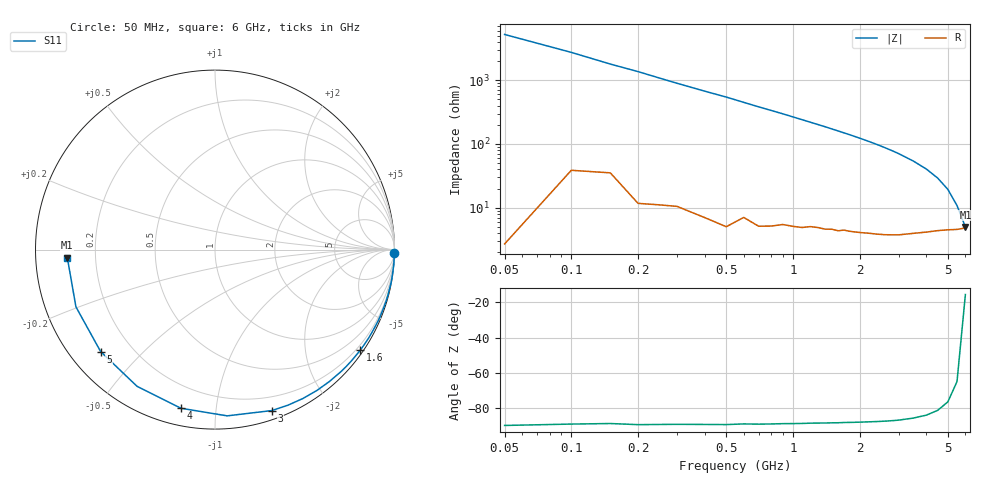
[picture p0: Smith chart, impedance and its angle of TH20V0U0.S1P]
! SIEMENS Discrete & RF Semiconductors
! BAS70
! Si Schottky Diode in SOT23
! VR = 20 V
! S-Parameters:  February  1997
# GHz  S  MA  R  50
!  f  S11
! GHz  MAG  ANG
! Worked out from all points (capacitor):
!   34 points, 50 MHz to 6 GHz, reference 50 ohm
!   read as one part to ground: C = 593 fF near 50 MHz
!   lowest |Z| = 5.01 ohm at 6 GHz (marker M1)
!   S11 on the Smith chart (normalised r, x): 50 MHz: open; 1.6 GHz: 0.09, -3.20; 3 GHz: 0.08, -1.41; 4 GHz: 0.08, -0.80; 5 GHz: 0.09, -0.38; 6 GHz: 0.10, -0.03
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0.05  1 -1.1
0.1  0.9995 -2.1
0.25  0.999 -5.3
0.3  0.9987 -6.4
0.4  0.9985 -8.5
0.5  0.9983 -10.5
0.7  0.9966 -14.9
0.8  0.9955 -17.0
0.9  0.994 -19.1
1  0.993 -21.3
1.1  0.9919 -23.5
1.2  0.99 -25.7
1.4  0.9876 -30.1
1.6  0.9846 -34.7
1.8  0.9808 -39.3
1.9  0.979 -41.7
2  0.9771 -44.1
2.2  0.9729 -49.0
2.4  0.9685 -54.1
2.6  0.9635 -59.4
2.8  0.9575 -64.9
3  0.9509 -70.6
3.5  0.9288 -85.8
4  0.904 -102.1
4.5  0.8768 -119.7
5  0.8536 -138.3
5.5  0.8379 -157.6
6  0.824 -176.9
